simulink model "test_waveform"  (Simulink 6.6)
settings: Solver=ode45  StartTime=0.0  StopTime=10.0  RelTol=1e-3
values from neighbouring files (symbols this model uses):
  param = params{get(handles.paramList, 'Value')}    [loopgui.m]
undefined symbols (not defined in the file or in its folder): param1, test_waveform
libraries: sltpda x9

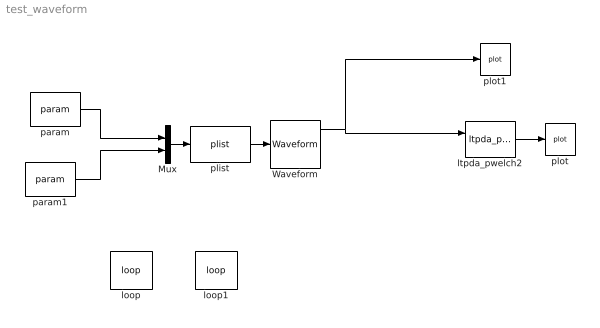
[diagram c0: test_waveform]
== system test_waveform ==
  Mux : Mux  Inputs=2
  Waveform : sltpda/Sources/Waveform  SystemSampleTime=-1  waveform=chirp  freq=0  phi=0  ntype=Normal  chirp_f0=1  chirp_fe=50  chirp_te=10  gp_f0=0  gp_bw=0  square_duty=0  sawtooth_width=0
  loop : sltpda/Parameters/loop  SystemSampleTime=-1  block=test_waveform/param  blockHandle=173.00146484375  key=val  vals=10 20 30  loopon=on
  loop1 : sltpda/Parameters/loop  SystemSampleTime=-1  block=test_waveform/param1  blockHandle=174.00146484375  key=val  vals=1000 2000  loopon=on
  ltpda_pwelch2 : sltpda/Signal Processing blocks/Frequency domain/ltpda_pwelch  Tag=ltpda_pwelch  Description=Makes a spectral density estimate by calling ltpda_pwlech.  SystemSampleTime=-1
  param : sltpda/Parameters/param  Tag=param  SystemSampleTime=-1  key=nsecs  val=10
  param1 : sltpda/Parameters/param  Tag=param  SystemSampleTime=-1  key=fs  val=1000
  plist : sltpda/Parameters/plist  SystemSampleTime=-1
  plot : sltpda/Sinks/plot  Tag=plot  Description=Plot an analysis object.  SystemSampleTime=-1  xscale=linear  yscale=linear
  plot1 : sltpda/Sinks/plot  Tag=plot  Description=Plot an analysis object.  SystemSampleTime=-1  xscale=linear  yscale=linear
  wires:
  param/1 -> Mux/1
  param1/1 -> Mux/2
  Mux/1 -> plist/1
  plist/1 -> Waveform/1
  ltpda_pwelch2/1 -> plot/1
  Waveform/1 -> plot1/1, ltpda_pwelch2/1
